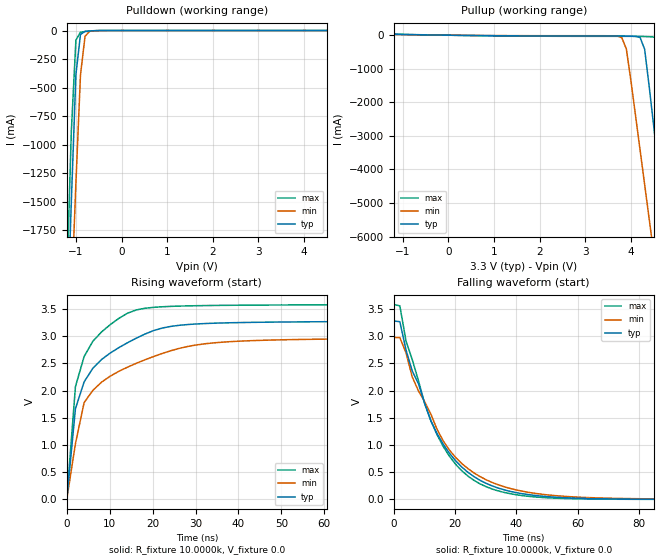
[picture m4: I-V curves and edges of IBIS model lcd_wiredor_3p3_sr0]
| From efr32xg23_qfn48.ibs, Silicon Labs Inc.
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|   Model lcd_wiredor_3p3_sr0
[Model]  lcd_wiredor_3p3_sr0
Model_type Output
Polarity   Non-Inverting
Enable   Active-Low
C_comp   1.6300pF   1.4000pF   2.7000pF
[Temperature Range]   25.0000   0.1250k   -40.0000
[Pullup Reference]   3.3000V   3.0000V   3.6000V
[Pulldown Reference]   0.0V   0.0V   0.0V
[POWER Clamp Reference]   3.3000V   3.0000V   3.6000V
[GND Clamp Reference]   0.0V   0.0V   0.0V
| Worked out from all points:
|   slope of the pullup table from 0 to 0.495 V, typ, clamps not added: 57.6 ohm
|   rising waveform, R_fixture 10.0000k, V_fixture 0.0: 20-80 % time 8.21ns typ, 11.6ns min, 5.08ns max; typ from 0 V to 3.28 V
|   falling waveform, R_fixture 10.0000k, V_fixture 0.0: 20-80 % time 16.4ns typ, 18.1ns min, 14.9ns max; typ from 3.28 V to 0 V
[Pulldown]
|Voltage   I(typ)   I(min)   I(max)
-3.3V     -27.87A    -25.05A    -30.64A
-1.2V     -2.686A    -3.389A    -2.22A
-1.1V     -1.495A    -2.361A    -881.8mA
-1V       -385.8mA   -1.337A    -84.19mA
-900mV    -35mA      -390.8mA   -14.95mA
-800mV    -7.709mA   -50.4mA    -8.405mA
-700mV    -3.744mA   -7.067mA   -4.22mA
-300mV    -2.853uA   -17.99uA   -699.1nA
6.6V      752.9nA    140.4uA    817.4nA
[Pullup]
|Voltage   I(typ)   I(min)   I(max)
-3.3V     128.6mA    111mA      144.8mA
3.8V      -24.76mA   -73.78mA   -32.98mA
3.9V      -26.81mA   -415.6mA   -32.99mA
4.3V      -417.3mA   -4.446A    -40.25mA
4.4V      -1.526A    -5.477A    -46.31mA
4.5V      -2.718A    -6.509A    -54.56mA
4.6V      -3.914A    -7.541A    -125mA
4.7V      -5.113A    -8.573A    -919.5mA
4.8V      -6.311A    -9.606A    -2.259A
5V        -8.709A    -11.67A    -4.955A
5.1V      -9.909A    -12.7A     -6.309A
6.6V      -27.92A    -28.2A     -26.63A
[Ramp]
| variable   typ   min   max
dV/dt_r  1.9690/8.2055n   1.7856/11.6366n   2.1507/5.0767n
dV/dt_f  60.0982u/2.1889p   67.7845u/4.0776p   84.5939u/0.6990n
R_load = 10.0000k
[Rising Waveform]
R_fixture= 10.0000k
V_fixture= 0.0
V_fixture_min= 0.0
V_fixture_max= 0.0
|time   V(typ)   V(min)   V(max)
0s        5.069uV    44.89uV    5.493uV
2.02ns    1.669V     1.024V     2.074V
4.04ns    2.16V      1.78V      2.627V
6.061ns   2.41V      2.003V     2.907V
8.081ns   2.571V     2.154V     3.078V
16.16ns   2.963V     2.501V     3.483V
24.24ns   3.182V     2.734V     3.55V
32.32ns   3.235V     2.863V     3.565V
44.44ns   3.257V     2.923V     3.573V
200ns     3.282V     2.976V     3.584V
[Falling Waveform]
R_fixture= 10.0000k
V_fixture= 0.0
V_fixture_min= 0.0
V_fixture_max= 0.0
|time   V(typ)   V(min)   V(max)
0s        3.283V     2.979V     3.586V
2.02ns    3.268V     2.977V     3.561V
4.04ns    2.747V     2.694V     2.912V
6.061ns   2.362V     2.252V     2.572V
10.1ns    1.768V     1.799V     1.765V
16.16ns   1.013V     1.074V     972.6mV
22.22ns   592.8mV    657.6mV    524.2mV
32.32ns   241mV      304.5mV    184.6mV
66.67ns   9.108mV    24mV       2.134mV
200ns     -487.9uV   162.9uV    -554.8uV
